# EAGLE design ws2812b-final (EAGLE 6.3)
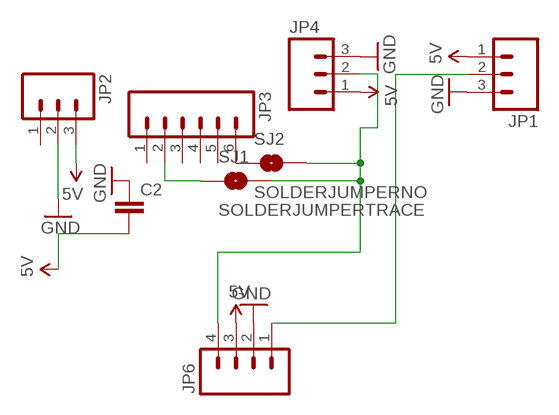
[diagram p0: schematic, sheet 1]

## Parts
C2  CAPPTH  [CAP-PTH-SMALL]
JP1  M03PTH  [1X03]
JP2  M03PTH  [1X03]
JP3  M06SIP  [1X06]
JP4  M03PTH  [1X03]
JP6  M041X04_NO_SILK  [1X04_NO_SILK]
SJ1  SOLDERJUMPERTRACE  [SJ_2S-TRACE]
SJ2  SOLDERJUMPERNO  [SJ_2S-NO]

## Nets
5V: C2.2 JP1.1 JP2.3 JP4.1 JP6.3
GND: C2.1 JP1.3 JP2.2 JP4.3 JP6.2
N$1: JP4.2 JP6.4 SJ1.2 SJ2.2
N$2: JP1.2 JP6.1
N$3: JP3.2 SJ1.1
N$4: JP3.6 SJ2.1
Unconnected: JP2.1 JP3.1 JP3.3 JP3.4 JP3.5

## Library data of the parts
C2 = SparkFun:CAP: Capacitor
JP1 JP4 = SparkFun-Connectors:M03: Header 3 Standard 3-pin 0.1" header. Use with straight break away headers (SKU : PRT-00116), right angle break away headers (PRT-00553), swiss pins (PRT-00743), machine pins (PRT-00117), and female headers (PRT-00115). Molex polarized connector foot print use with SKU : PRT-08232 with associated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
JP2 = SparkFun:M03: Header 3 Standard 3-pin 0.1" header. Use with straight break away headers (SKU : PRT-00116), right angle break away headers (PRT-00553), swiss pins (PRT-00743), machine pins (PRT-00117), and female headers (PRT-00115). Molex polarized connector foot print use with SKU : PRT-08232 with associated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
JP3 = SparkFun:M06: Header 6 Standard 6-pin 0.1" header. Use with straight break away headers (SKU : PRT-00116), right angle break away headers (PRT-00553), swiss pins (PRT-00743), machine pins (PRT-00117), and female headers (PRT-00115). Molex polarized connector foot print use with SKU : PRT-08094 with associated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
JP6 = Digistump:M04: Header 4 Standard 4-pin 0.1" header. Use with straight break away headers (SKU : PRT-00116), right angle break away headers (PRT-00553), swiss pins (PRT-00743), machine pins (PRT-00117), and female headers (PRT-00115). Molex polarized connector foot print use with SKU : PRT-08231 with associated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
SJ1 SJ2 = SparkFun-Passives:SOLDERJUMPER: Solder Jumper

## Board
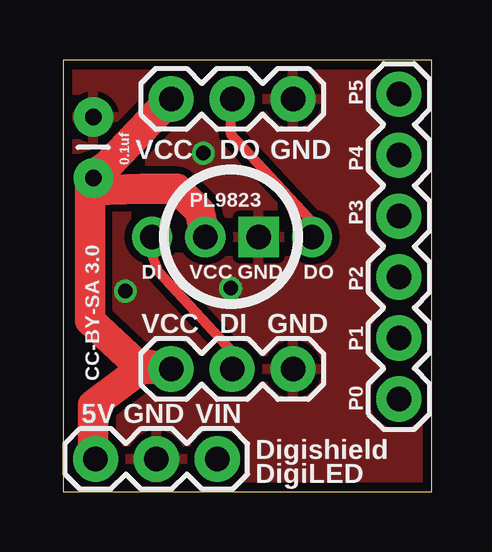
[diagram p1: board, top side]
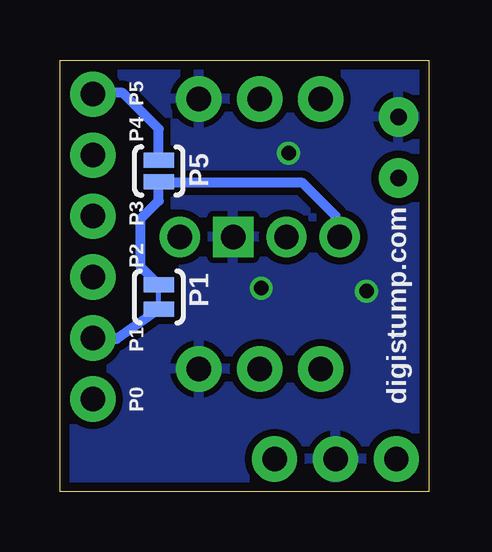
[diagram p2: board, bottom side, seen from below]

Size 15.38 x 17.99 mm. Coordinates in mm from the lower left corner, seen from the top.
Outline: 0,17.99 0,0 15.38,0 15.38,17.99 0,17.99
Copper layers (1*16): Top 0.0356mm / dielectric 1.5011mm / Bottom 0.0356mm
Design rules "default *": minimum track width 8mil, minimum drill 13mil, track to track 12mil, track to pad 12mil, pad to pad 12mil, via to via 12mil, smd to smd 8mil, copper to edge 15mil, drill to drill 12mil, minimum pad ring 7mil, minimum via ring 7mil, stop-mask expansion 4mil, vias tented up to drill 50mil, thermal gap 10mil

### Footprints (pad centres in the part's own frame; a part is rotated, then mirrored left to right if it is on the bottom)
CAP-PTH-SMALL = drill 0.7 pad 1.651: 1 0,0; 2 2.54,0
1X03 = drill 1.016 pad 1.88: 1 0,0; 2 2.54,0; 3 5.08,0
1X06 = drill 1.016 pad 1.88: 1 0,0; 2 2.54,0; 3 5.08,0; 4 7.62,0; 5 10.16,0; 6 12.7,0
1X04_NO_SILK = drill 1.016 pad 1.676: 1 0,0; 3 4.445,0; 4 6.668,0 | drill 1.016 pad 1.676 square: 2 2.223,0
SJ_2S-TRACE = smd 0.635 x 1.27: 1 -0.508,0; 2 0.508,0
SJ_2S-NO = smd 0.635 x 1.27: 1 -0.45,0; 2 0.45,0

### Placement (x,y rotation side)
C2  1.25,15.62 270 top
JP1  4.5,16.37 0 top
JP2  6.42,1.37 180 top
JP3  14,3.87 90 top
JP4  4.5,5.12 0 top
JP6  10.37,10.62 180 top
SJ1  11.25,8.12 90 bottom
SJ2  11.25,13.37 270 bottom

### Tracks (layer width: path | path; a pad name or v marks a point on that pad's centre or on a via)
5V
  Top 0.406: C2.2 1.17,13.08 1.13,13.12
  Top 0.813: 1,12.32 1.25,12.57
  Top 1.27: JP2.3 1.25,1.46 1.25,3.62 3.25,5.12 JP4.1 3,5.37 1.13,7.12 1.13,12.62 | 1.13,12.62 1.13,13.12 1.88,13.62 JP1.1 | 1.13,12.62 1.55,12.57 1.25,12.57 3.3,12.62 4.75,12.62 5.67,11.7 JP6.3
GND  (via drill 0.6)
  other vias: 5.84,14.11 2.59,8.36 6.98,8.48
  pour Top: 0,17.87 0,0.12 15.25,0.12 15.25,17.87
  pour Bottom: 0,17.87 0,0.12 15.25,0.12 15.25,17.87
N$1
  Top 0.406: JP4.2 7.04,5.83 4,9.12 3.75,9.75 JP6.4
  Bottom 0.406: SJ1.2 12,9.38 12,11.37 11.25,12.12 SJ2.2 10.95,12.87 5.25,12.87 3.88,11.5 JP6.4
N$2
  Top 0.406: JP6.1 10.25,11.37 7,14.87 7,16.33 JP1.2
N$3
  Bottom 0.406: JP3.2 12.96,6.41 13,6.37 SJ1.1
N$4
  Bottom 0.406: SJ2.1 11.25,15.12 12.75,16.62 13.95,16.62 JP3.6

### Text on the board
tPlace: 0.1uf | VCC | DO | GND | PL9823 | DI | VCC | GND | DO | VCC | DI | GND | CC-BY-SA 3.0 | 5V | GND | VIN | Digishield | DigiLED
bPlace: P5 | digistump.com | P1
tNames: P5 | P4 | P3 | P2 | P1 | P0
bNames: P5 | P4 | P3 | P2 | P1 | P0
